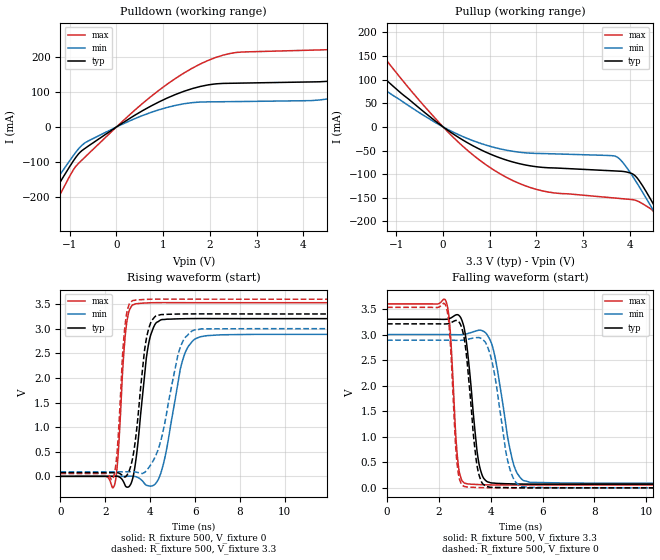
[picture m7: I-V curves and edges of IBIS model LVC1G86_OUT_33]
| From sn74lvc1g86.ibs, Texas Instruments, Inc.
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[Model]   LVC1G86_OUT_33
Model_type  Output
Vref =   0
Rref =   500
Cref =   50p
Vmeas =   1.5
| variable   typ   min   max
C_comp   9.41pF   5.87pF   12.64pF
| C_pullup   9.59pF   5.87pF   11.73pF
| C_pulldown   9.23pF   6.36pF   12.64pF
[Temperature Range]   40   100   -40
| Ambient temperature   25   85   -40
[Voltage range]   3.3   3   3.6
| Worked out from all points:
|   slope of the pulldown table from 0 to 0.495 V, typ, clamps not added: 11.9 ohm
|   slope of the pullup table from 0 to 0.495 V, typ, clamps not added: 15.5 ohm
|   rising waveform, R_fixture 500, V_fixture 0: 20-80 % time 437ps typ, 672ps min, 272ps max; typ from 0 V to 3.21 V
|   falling waveform, R_fixture 500, V_fixture 3.3: 20-80 % time 363ps typ, 558ps min, 227ps max; typ from 3.3 V to 0.073 V
|   rising waveform, R_fixture 500, V_fixture 3.3: 20-80 % time 443ps typ, 774ps min, 272ps max; typ from 0.073 V to 3.3 V
|   falling waveform, R_fixture 500, V_fixture 0: 20-80 % time 348ps typ, 521ps min, 220ps max; typ from 3.21 V to 0 V
[Pulldown]
| LVC1G86_OUT_33
|   Voltage   I(typ)   I(min)   I(max)
-5V       -987.4mA   -880.3mA   -1.157A
-2.035V   -343.4mA   -301.4mA   -410.2mA
-1.495V   -222mA     -193.1mA   -268.4mA
-580mV    -52.55mA   -38.35mA   -74.1mA
1.085V    82.51mA    55.72mA    122.1mA
2.285V    124.4mA    72.05mA    205.2mA
4.935V    138.4mA    90.07mA    223.9mA
6.945V    245mA      178mA      348.6mA
7.505V    285.4mA    89.25mA    403.3mA
7.92V     300mA      81.48mA    446.9mA
8.75V     157.7mA    82.47mA    508.5mA
10V       144.2mA    84.07mA    275.5mA
[Pullup]
| LVC1G86_OUT_33
|   Voltage   I(typ)   I(min)   I(max)
-5V       489.6mA    392.1mA    680.3mA
-2.855V   258.7mA    204.1mA    363.3mA
-2.31V    203.4mA    159.5mA    286.8mA
-1.81V    154.5mA    120.3mA    218.8mA
-35mV     2.551mA    1.908mA    3.712mA
1.015V    -57.68mA   -41.29mA   -86.63mA
2.125V    -85.61mA   -56.32mA   -135.3mA
3.7V      -93.27mA   -62.52mA   -150.7mA
4.12V     -104.2mA   -113.9mA   -155.3mA
4.465V    -156.8mA   -170.6mA   -174.9mA
4.725V    -203.6mA   -215.5mA   -217.7mA
10V       -1.272A    -1.208A    -1.41A
[Ramp]
| LVC1G86_OUT_33
| variable   typ   min   max
dV/dt_r   2.05/4.90E-10   1.85/7.58E-10   2.25/2.96E-10
dV/dt_f   1.99/3.88E-10   1.80/6.12E-10   2.18/2.43E-10
R_load = 500
[Rising Waveform]
| LVC1G86_OUT_33
R_fixture =   500
C_fixture =   0
L_fixture =   0
V_fixture =   0
V_fixture_min = 0
V_fixture_max = 0
|   Time   V(typ)   V(min)   V(max)
0s        146.9pV    5.25nV     591.7pV
2.39ns    1.727mV    -73.42uV   -200.4mV
2.56ns    -211.1uV   -47.19uV   382.9mV
2.925ns   -211.2mV   1.182mV    3.026V
3.37ns    362.7mV    -9.056mV   3.508V
3.92ns    2.672V     -191mV     3.526V
4.535ns   3.187V     159.7mV    3.531V
5.5ns     3.204V     2.441V     3.53V
6.54ns    3.206V     2.86V      3.529V
50ns      3.205V     2.883V     3.529V
[Falling Waveform]
| LVC1G86_OUT_33
R_fixture =   500
C_fixture =   0
L_fixture =   0
V_fixture =   3.3
V_fixture_min = 3
V_fixture_max = 3.6
|   Time   V(typ)   V(min)   V(max)
0s        3.3V       3V         3.6V
2.265ns   3.299V     3V         3.662V
2.435ns   3.318V     2.999V     3.088V
2.745ns   3.385V     2.996V     460.1mV
3.11ns    2.648V     3.019V     76.8mV
3.695ns   215.5mV    3.07V      60.6mV
4.13ns    92.59mV    2.642V     56.44mV
4.89ns    76.52mV    445.7mV    55.34mV
5.535ns   72.51mV    107.3mV    55.55mV
50ns      72.53mV    91.16mV    55.91mV
[Rising Waveform]
| LVC1G86_OUT_33
R_fixture =   500
C_fixture =   0
L_fixture =   0
V_fixture =   3.3
V_fixture_min = 3
V_fixture_max = 3.6
|   Time   V(typ)   V(min)   V(max)
0s        72.51mV    91.13mV    55.9mV
2.34ns    73.51mV    91.07mV    -45.67mV
2.53ns    75.14mV    91.08mV    530.9mV
2.875ns   -12.93mV   91.97mV    3.054V
3.25ns    453.2mV    93.43mV    3.576V
3.845ns   2.836V     121.9mV    3.596V
4.48ns    3.287V     739.9mV    3.601V
5.345ns   3.299V     2.626V     3.601V
6.28ns    3.301V     2.998V     3.6V
50ns      3.3V       3V         3.6V
[Falling Waveform]
| LVC1G86_OUT_33
R_fixture =   500
C_fixture =   0
L_fixture =   0
V_fixture =   0
V_fixture_min = 0
V_fixture_max = 0
|   Time   V(typ)   V(min)   V(max)
0s        3.209V     2.89V      3.532V
2.255ns   3.208V     2.889V     3.579V
2.415ns   3.222V     2.889V     3.029V
2.71ns    3.274V     2.887V     434.2mV
3.075ns   2.535V     2.902V     16.88mV
3.64ns    120.5mV    2.921V     4.022mV
4.06ns    9.364mV    2.448V     554.2uV
4.74ns    3.362mV    364.5mV    -481.4uV
5.39ns    86.6uV     11.48mV    -292.8uV
50ns      18.15uV    28.39uV    11.12uV
